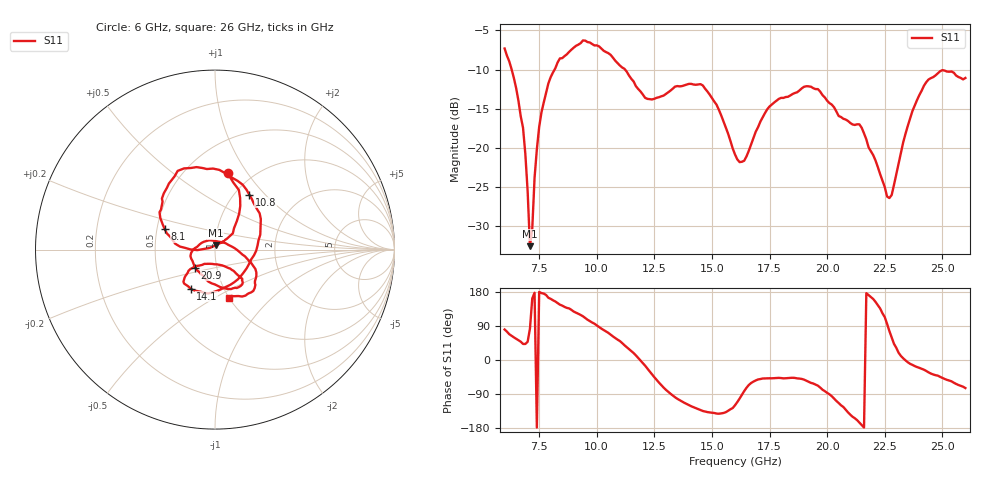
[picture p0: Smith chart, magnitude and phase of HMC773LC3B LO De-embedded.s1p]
! Hittite Microwave Corporation
! 20 Alpha Road
! Chelmsford, MA 01824
! http://www.hittite.com
! Tel: 978-250-3343
! Fax: 978-250-3373
! Device:  HMC773LC3B
! Description: GaAS MMIC Fundamental Mixer
! Frequency:  6-  26 GHz Mixer
! Package:  LC3B - 3x3 mm QFN Ceramic High frequency SMT Package: 12 pin
! Ports
!  Pin  2  = LO
!  Pin  5  = IF
!  pin  8  = RF
! Data:  The device was measured on evaluation board 125040-1.
!  The evaluation circuit board was modeled and simulated.  This was use
!  to removed the evaluation board circuit from the measured data.
!  The reference plane is the center of the package pin.
! Misc:
! Date Measured:  09-10-2009
! Date:  09-10-2009
! Note:
!  Hittite supplies this data as a sample of measured data at the package pin for
!  for this package product.  Your particular data for this product may vary.
!  Data was taken at 25 degrees C.
!  Hittite reserves the right to change this data at anytime.
# MHz S MA R 50
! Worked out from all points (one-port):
!   201 points, 6 GHz to 26 GHz, reference 50 ohm
!   lowest |S11| = -32.5 dB at 7.1 GHz (marker M1), VSWR 1.05, Z = 50.2 + j2.36 ohm
!   |S11| at or under -10 dB: 6.308 GHz to 8.168 GHz (1.861 GHz wide, 25.7 % of centre); 11.23 GHz to end of sweep
!   S11 on the Smith chart (normalised r, x): 6 GHz: 0.78, +0.82; 8.1 GHz: 0.55, +0.14; 10.8 GHz: 1.16, +0.82; 14.1 GHz: 0.70, -0.33; 20.9 GHz: 0.79, -0.16; 26 GHz: 1.00, -0.58
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6000  0.4312 80.5
6800  0.1345 42.3
7000  0.05301 48.1
7100  0.02369 82.8
7200  0.0306 162.3
7300  0.0645 177.4
7500  0.1363 179.7
8100  0.3035 157.6
8500  0.3744 143.6
9500  0.484 110.9
10800  0.3609 58.0
11000  0.3364 50.1
12200  0.2059 -22.5
13500  0.2484 -102.5
14100  0.2566 -122.0
15200  0.1889 -141.3
16000  0.09107 -119.5
16400  0.08306 -82.0
17400  0.1768 -48.6
18500  0.2211 -46.9
19600  0.2376 -67.8
20900  0.149 -137.9
21000  0.1447 -144.1
21500  0.1346 -171.8
22700  0.04802 76.5
23500  0.1385 -5.9
24400  0.2736 -32.6
26000  0.2798 -74.1
